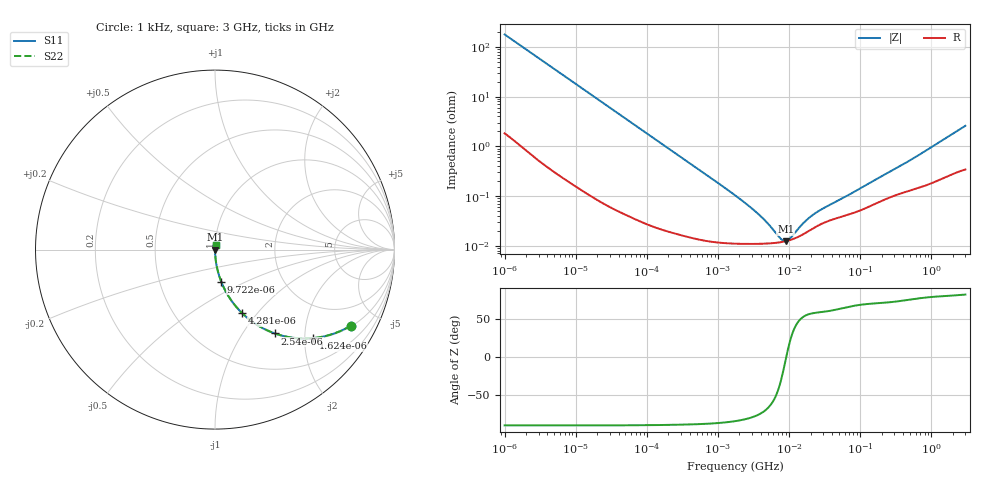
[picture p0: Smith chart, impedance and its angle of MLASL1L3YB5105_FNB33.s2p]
! MLASL1L3YB5105_FNB33  S-PARAMETER MODEL  ( Standard Model )
! Model Generated by TAIYO YUDEN Corporation (http://www.ty-top.com)
! Version 1.0
! TAIYO YUDEN Control No. 220601
! Copyright(c) 2012 TAIYO YUDEN CO.,LTD. All Rights Reserved.
! Product Description (link to TY-COMPAS)
! https://ds.yuden.co.jp/TYCOMPAS/or/detail?pn=MLASL1L3YB5105KFNB33&u=M
! Products Name : Multilayer Ceramic Capacitors
! Characteristics :
!  Capacitance : 1 [uF] , Rated Voltage : 10 [V] , TCC : X5R
!  Case Size : 1.0 x 0.5 / 0.039 x 0.02 [mm/inch] , Thickness : 0.3 / 0.012 [mm/inch]
!  (Conditions: Temperature = 25 [degC] , DC Bias Voltage = 0 [V])
! External Node Assignments :
!  1  o---| |---o  2
! GND o---------o GND
! Frequency Range : 1kHz  -  3GHz  [ 401 STEP ]
# MHZ S RI R 50
! Freq[MHz].  S11 Real  S11 Imag  S21 Real  S21 Imag  S12 Real  S12 Imag  S22 Real  S22 Imag
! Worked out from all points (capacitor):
!   401 points, 1 kHz to 3 GHz, reference 50 ohm
!   read as one part in series: C = 892 nF near 1.077 kHz
!   lowest |Z| = 12.3 mohm at 8.934 MHz (marker M1)
!   series resonance near 9.081 MHz, so ESL is about 340 pH
!   S11 on the Smith chart (normalised r, x): 1 kHz: 1.04, -3.56; 1.624 kHz: 1.02, -2.20; 2.54 kHz: 1.01, -1.41; 4.281 kHz: 1.01, -0.84; 9.722 kHz: 1.00, -0.37; 3 GHz: 1.01, +0.05
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0.001  0.7579 -0.4233  0.2421 0.4233  0.2421 0.4233  0.7579 -0.4233
0.001624  0.5473 -0.493  0.4527 0.493  0.4527 0.493  0.5473 -0.493
0.00254  0.3336 -0.4671  0.6664 0.4671  0.6664 0.4671  0.3336 -0.4671
0.004281  0.1518 -0.3546  0.8482 0.3546  0.8482 0.3546  0.1518 -0.3546
0.006215  0.0792 -0.2659  0.9208 0.2659  0.9208 0.2659  0.0792 -0.2659
0.009722  0.0347 -0.1787  0.9653 0.1787  0.9653 0.1787  0.0347 -0.1787
0.01216  0.0228 -0.1449  0.9772 0.1449  0.9772 0.1449  0.0228 -0.1449
0.033275  0.00351 -0.0543  0.9965 0.0543  0.9965 0.0543  0.00351 -0.0543
0.147855  0.000373 -0.0124  0.9996 0.0124  0.9996 0.0124  0.000373 -0.0124
1.732051  0.000111 -0.00103  0.9999 0.00103  0.9999 0.00103  0.000111 -0.00103
3.651041  0.000109 -0.000426  0.9999 0.000426  0.9999 0.000426  0.000109 -0.000426
4.919932  0.000111 -0.000267  0.9999 0.000267  0.9999 0.000267  0.000111 -0.000267
7.414467  0.000117 -8.36e-05  0.9999 8.36e-05  0.9999 8.36e-05  0.000117 -8.36e-05
8.291982  0.00012 -3.72e-05  0.9999 3.72e-05  0.9999 3.72e-05  0.00012 -3.72e-05
8.933959  0.000123 -6.6e-06  0.9999 6.6e-06  0.9999 6.6e-06  0.000123 -6.6e-06
10.37087  0.00013 5.43e-05  0.9999 -5.43e-05  0.9999 -5.43e-05  0.00013 5.43e-05
15.62917  0.000169 0.000223  0.9998 -0.000223  0.9998 -0.000223  0.000169 0.000223
21.06097  0.000218 0.000345  0.9998 -0.000345  0.9998 -0.000345  0.000218 0.000345
29.45871  0.000282 0.000479  0.9997 -0.000479  0.9997 -0.000479  0.000282 0.000479
256.0921  0.000937 0.00289  0.9991 -0.00289  0.9991 -0.00289  0.000937 0.00289
560.3316  0.00138 0.00559  0.9986 -0.00559  0.9986 -0.00559  0.00138 0.00559
3000  0.00407 0.0255  0.9959 -0.0255  0.9959 -0.0255  0.00407 0.0255
